TYPE Info :
STRUCT
	Warning:Warning;
	Alarm:Alarm;
	
	//Tolerance	
	(*PRESSURE_Warning:BOOL;
	PRESSURE_Alarm:BOOL;
	
	MFC1_Warning:BOOL;
	MFC1_Alarm:BOOL;
	
	MFC2_Warning:BOOL;
	MFC2_Alarm:BOOL;
	
	MFC3_Warning:BOOL;
	MFC3_Alarm:BOOL;
	
	MFC4_Warning:BOOL;
	MFC4_Alarm:BOOL;
	
	MFC5_Warning:BOOL;
	MFC5_Alarm:BOOL;
	
	MFC6_Warning:BOOL;
	MFC6_Alarm:BOOL;
	
	MFC7_Warning:BOOL;
	MFC7_Alarm:BOOL;
	
	MFC8_Warning:BOOL;
	MFC8_Alarm:BOOL;
	
	MFC9_Warning:BOOL;
	MFC9_Alarm:BOOL;
	
	WALL_TEMP_Warning:BOOL;
	WALL_TEMP_Alarm:BOOL;
	
	LID_TEMP_Warning:BOOL;
	LID_TEMP_Alarm:BOOL;
	
	STAGE_EDGE_TEMP_Warning:BOOL;
	STAGE_EDGE_TEMP_Alarm:BOOL;
	
	STAGE_CENTER_TEMP_Warning: BOOL;
	STAGE_CENTER_TEMP_ALARM: BOOL;
	*)

	
	(*//
	ALARM_PLC:BOOL;	
	ALARM_DRY_PUMP:BOOL;
	ALARM_PENDULUM_VALVE:BOOL;
	ALARM_TURBO_PUMP:BOOL;
	ALARM_CHILLER1:BOOL;
	ALARM_CHILLER2:BOOL;

	WARNING_CHILLER1:BOOL;
	WARNING_CHILLER2:BOOL;
	*)
	
	
	
	
	
	
	
	
	
	
	
	
	
	
	
	
	
	
	
	
	
	
	
	
	
	
	
	
	
	
	
	
	
	
	
	
	
END_STRUCT
END_TYPE
